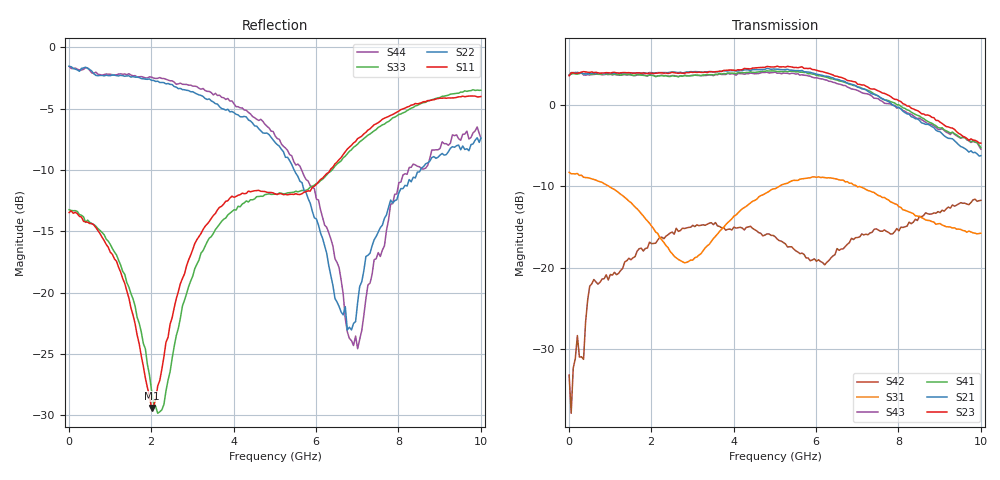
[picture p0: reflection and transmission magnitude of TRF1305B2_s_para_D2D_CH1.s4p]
! Created Thu Apr 18 16:54:47 2024
# hz S ri R 50
! 4 Port Network Data from SP1.SP block
!port1 - INP, port2 - OUTP, port3 - INM, port4 - OUTM
! freq  reS11  imS11  reS12  imS12  reS13  imS13  reS14  imS14
!  reS21  imS21  reS22  imS22  reS23  imS23  reS24  imS24
!  reS31  imS31  reS32  imS32  reS33  imS33  reS34  imS34
!  reS41  imS41  reS42  imS42  reS43  imS43  reS44  imS44
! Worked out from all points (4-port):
!   201 points, 10 MHz to 10 GHz, reference 50 ohm
!   strongest paths, dB at 10 MHz, 2.51 GHz, 5.01 GHz, 7.51 GHz, 10 GHz:
!     S23: 3.6, 4.0, 4.7, 1.7, -4.7
!     S21: 3.6, 4.1, 4.4, 1.1, -6.2
!     S41: 3.7, 3.6, 4.2, 1.1, -5.3
!     S43: 3.7, 3.6, 4.0, 0.8, -5.4
!     S31: -8.3, -18.3, -10.3, -11.1, -15.8
!     S42: -33.2, -15.6, -16.2, -15.4, -11.7
!   lowest |S11| = -29.4 dB at 2.01 GHz (marker M1), VSWR 1.07, Z = 53.5 - j0.458 ohm
!   |S11| at or under -10 dB: start of sweep to 6.345 GHz
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1e7  0.2121 -0.00151  0.00389 0.0139  0.3803 -0.00339  0.0129 0.00248
     1.52 0.00154  -0.8356 -0.0128  -1.512 0.00991  -0.0285 -0.00503
     0.3847 -0.00159  -0.000447 -0.000232  0.2175 0.00952  0.0106 0.0103
     -1.524 -0.0235  -0.02 0.00886  1.524 0.0299  -0.837 0.0215
1.6e8  0.2115 -0.0222  0.00137 0.00672  0.377 -0.049  0.00341 0.00631
       1.565 -0.1629  -0.8133 0.039  -1.551 0.1713  0.0167 0.0283
       0.3734 -0.05  0.00734 0.00863  0.2146 -0.0228  0.00206 0.00556
       -1.541 0.1774  0.00869 0.0261  1.575 -0.1732  -0.8222 0.0367
2.01e9  0.0336 -0.00427  0.0329 -0.00481  -0.027 -0.185  0.0443 0.00504
        0.3178 -1.546  -0.6982 0.2221  -0.2087 1.555  0.1287 0.0544
        -0.0317 -0.177  0.0467 0.0055  0.0337 -0.0212  0.0306 -0.00492
        -0.1953 1.507  0.1332 0.0439  0.2857 -1.498  -0.7095 0.2597
4.26e9  0.2403 0.0789  -0.0105 -0.0438  0.037 0.2452  0.038 -0.0544
        -1.618 -0.2784  -0.417 0.3151  1.667 0.1822  0.1191 -0.1417
        0.0516 0.2277  0.0397 -0.058  0.2172 0.0821  -0.0101 -0.0427
        1.569 0.16  0.1137 -0.1268  -1.519 -0.2756  -0.4183 0.3646
5.86e9  0.257 0.0339  -0.0306 0.000813  0.3582 0.1253  -0.0111 -0.0813
        -0.6366 1.452  -0.1332 0.1893  0.5698 -1.579  -0.0818 -0.0401
        0.3347 0.1218  -0.00716 -0.0845  0.2691 0.0108  -0.0291 -0.00287
        0.5433 -1.462  -0.091 -0.0621  -0.6458 1.355  -0.1406 0.234
7.81e9  0.4973 -0.1774  0.00097 -0.000716  0.2086 -0.1254  -0.0786 -0.0415
        0.9835 0.2967  -0.1775 -0.1591  -1.073 -0.3422  0.0158 0.1752
        0.2222 -0.1216  -0.0796 -0.0496  0.4619 -0.2063  0.00129 0.00472
        -0.9836 -0.3614  -0.00268 0.1606  0.9224 0.4194  -0.1026 -0.2052
1e10  0.1618 -0.6086  -0.0225 -0.000909  0.1247 -0.1129  -0.0749 0.0548
      0.1831 -0.452  -0.3779 -0.1974  -0.2654 0.5174  0.1861 0.2331
      0.119 -0.1108  -0.088 0.0521  0.1125 -0.6585  -0.0139 -0.00272
      -0.2816 0.468  0.1312 0.2232  0.2474 -0.4738  -0.3476 -0.2476
